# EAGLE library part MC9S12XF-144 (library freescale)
MC9S12XF512 Source: www.freescale.com .. MC9S12XF512V1RM.pdf
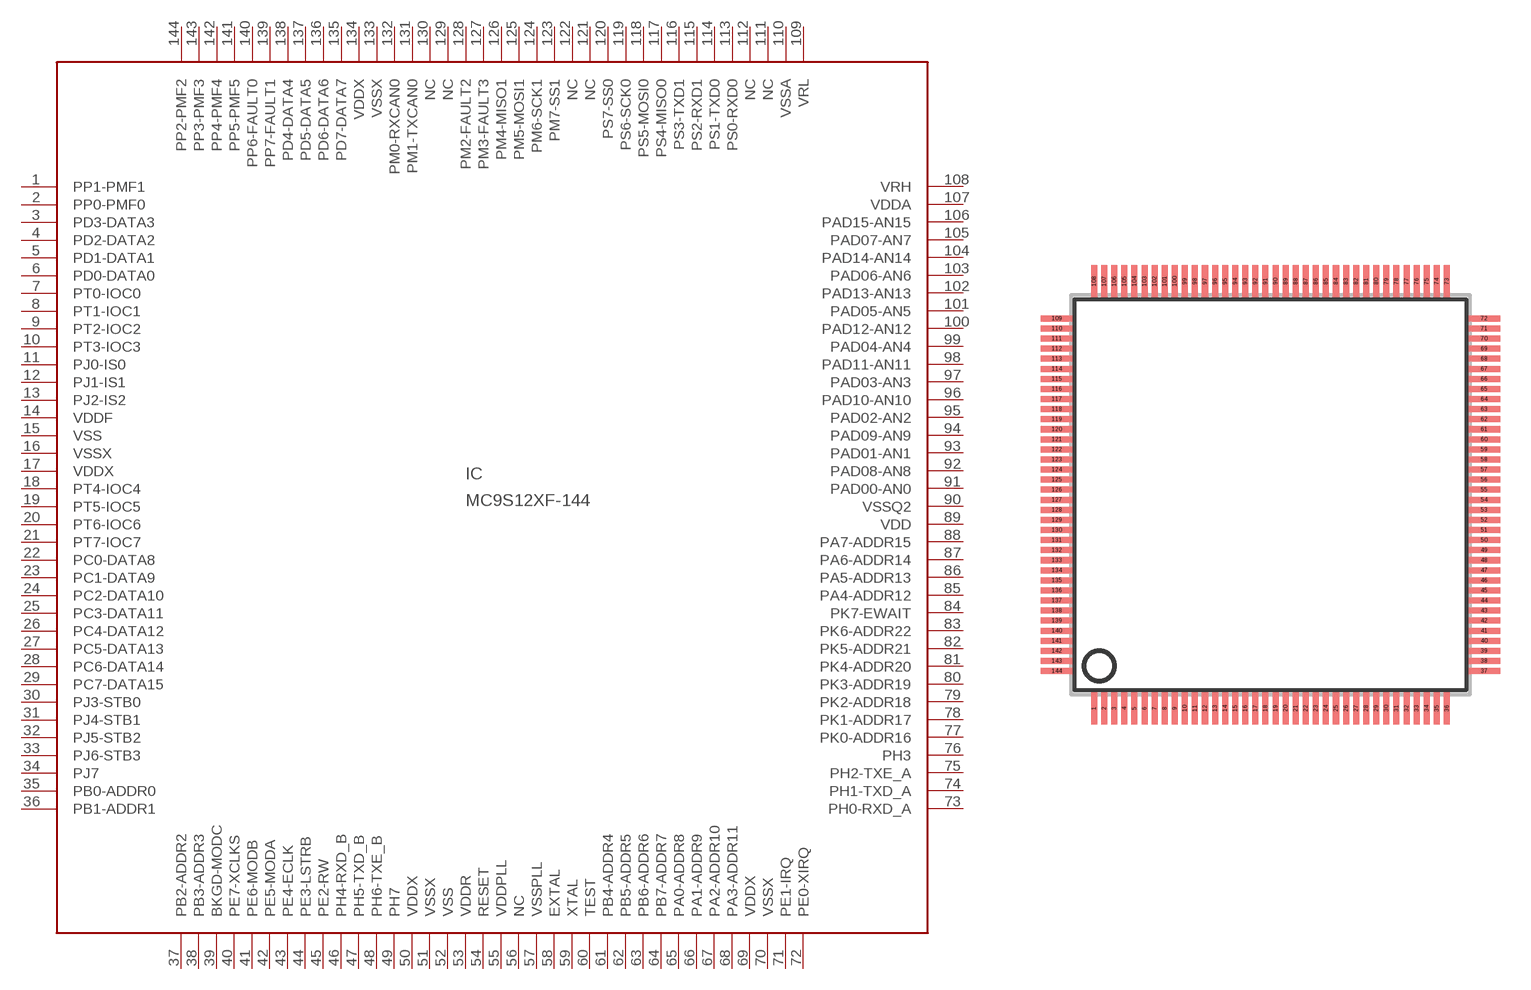
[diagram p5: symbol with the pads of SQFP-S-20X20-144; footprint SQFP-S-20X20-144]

Designator prefix IC

## MC9S12XF-144 (MPN: LFDAS12XFLT; OC_FARNELL: unknown; OC_NEWARK: 14M5920)  [SQFP-S-20X20-144]
1  PP1-PMF1
2  PP0-PMF0
3  PD3-DATA3
4  PD2-DATA2
5  PD1-DATA1
6  PD0-DATA0
7  PT0-IOC0
8  PT1-IOC1
9  PT2-IOC2
10  PT3-IOC3
11  PJ0-IS0
12  PJ1-IS1
13  PJ2-IS2
14  VDDF  pwr
15  VSS  pwr
16  VSSX  pwr
17  VDDX  pwr
18  PT4-IOC4
19  PT5-IOC5
20  PT6-IOC6
21  PT7-IOC7
22  PC0-DATA8
23  PC1-DATA9
24  PC2-DATA10
25  PC3-DATA11
26  PC4-DATA12
27  PC5-DATA13
28  PC6-DATA14
29  PC7-DATA15
30  PJ3-STB0
31  PJ4-STB1
32  PJ5-STB2
33  PJ6-STB3
34  PJ7
35  PB0-ADDR0
36  PB1-ADDR1
37  PB2-ADDR2
38  PB3-ADDR3
39  BKGD-MODC
40  PE7-XCLKS
41  PE6-MODB
42  PE5-MODA
43  PE4-ECLK
44  PE3-LSTRB
45  PE2-RW
46  PH4-RXD_B
47  PH5-TXD_B
48  PH6-TXE_B
49  PH7
50  VDDX  pwr
51  VSSX  pwr
52  VSS  pwr
53  VDDR  pwr
54  RESET
55  VDDPLL  pwr
56  NC  nc
57  VSSPLL  pwr
58  EXTAL  pas
59  XTAL  pas
60  TEST  in
61  PB4-ADDR4
62  PB5-ADDR5
63  PB6-ADDR6
64  PB7-ADDR7
65  PA0-ADDR8
66  PA1-ADDR9
67  PA2-ADDR10
68  PA3-ADDR11
69  VDDX  pwr
70  VSSX  pwr
71  PE1-IRQ  in
72  PE0-XIRQ  in
73  PH0-RXD_A
74  PH1-TXD_A
75  PH2-TXE_A
76  PH3
77  PK0-ADDR16
78  PK1-ADDR17
79  PK2-ADDR18
80  PK3-ADDR19
81  PK4-ADDR20
82  PK5-ADDR21
83  PK6-ADDR22
84  PK7-EWAIT
85  PA4-ADDR12
86  PA5-ADDR13
87  PA6-ADDR14
88  PA7-ADDR15
89  VDD  pwr
90  VSSQ2  pwr
91  PAD00-AN0
92  PAD08-AN8
93  PAD01-AN1
94  PAD09-AN9
95  PAD02-AN2
96  PAD10-AN10
97  PAD03-AN3
98  PAD11-AN11
99  PAD04-AN4
100  PAD12-AN12
101  PAD05-AN5
102  PAD13-AN13
103  PAD06-AN6
104  PAD14-AN14
105  PAD07-AN7
106  PAD15-AN15
107  VDDA  pwr
108  VRH  pwr
109  VRL  pwr
110  VSSA  pwr
111  NC  nc
112  NC  nc
113  PS0-RXD0
114  PS1-TXD0
115  PS2-RXD1
116  PS3-TXD1
117  PS4-MISO0
118  PS5-MOSI0
119  PS6-SCK0
120  PS7-SS0
121  NC  nc
122  NC  nc
123  PM7-SS1
124  PM6-SCK1
125  PM5-MOSI1
126  PM4-MISO1
127  PM3-FAULT3
128  PM2-FAULT2
129  NC  nc
130  NC  nc
131  PM1-TXCAN0
132  PM0-RXCAN0
133  VSSX  pwr
134  VDDX  pwr
135  PD7-DATA7
136  PD6-DATA6
137  PD5-DATA5
138  PD4-DATA4
139  PP7-FAULT1
140  PP6-FAULT0
141  PP5-PMF5
142  PP4-PMF4
143  PP3-PMF3
144  PP2-PMF2

## Footprint SQFP-S-20X20-144 (pad centres in mm)
QFP144 shrink quad flat pack, square
smd 0.3 x 1.6: 1 -8.75,-10.6; 2 -8.25,-10.6; 3 -7.75,-10.6; 4 -7.25,-10.6; 5 -6.75,-10.6; 6 -6.25,-10.6; 7 -5.75,-10.6; 8 -5.25,-10.6; 9 -4.75,-10.6; 10 -4.25,-10.6; 11 -3.75,-10.6; 12 -3.25,-10.6; 13 -2.75,-10.6; 14 -2.25,-10.6; 15 -1.75,-10.6; 16 -1.25,-10.6; 17 -0.75,-10.6; 18 -0.25,-10.6; 19 0.25,-10.6; 20 0.75,-10.6; 21 1.25,-10.6; 22 1.75,-10.6; 23 2.25,-10.6; 24 2.75,-10.6; 25 3.25,-10.6; 26 3.75,-10.6; 27 4.25,-10.6; 28 4.75,-10.6; 29 5.25,-10.6; 30 5.75,-10.6; 31 6.25,-10.6; 32 6.75,-10.6; 33 7.25,-10.6; 34 7.75,-10.6; 35 8.25,-10.6; 36 8.75,-10.6; 73 8.75,10.6; 74 8.25,10.6; 75 7.75,10.6; 76 7.25,10.6; 77 6.75,10.6; 78 6.25,10.6; 79 5.75,10.6; 80 5.25,10.6; 81 4.75,10.6; 82 4.25,10.6; 83 3.75,10.6; 84 3.25,10.6; 85 2.75,10.6; 86 2.25,10.6; 87 1.75,10.6; 88 1.25,10.6; 89 0.75,10.6; 90 0.25,10.6; 91 -0.25,10.6; 92 -0.75,10.6; 93 -1.25,10.6; 94 -1.75,10.6; 95 -2.25,10.6; 96 -2.75,10.6; 97 -3.25,10.6; 98 -3.75,10.6; 99 -4.25,10.6; 100 -4.75,10.6; 101 -5.25,10.6; 102 -5.75,10.6; 103 -6.25,10.6; 104 -6.75,10.6; 105 -7.25,10.6; 106 -7.75,10.6; 107 -8.25,10.6; 108 -8.75,10.6
smd 1.6 x 0.3: 37 10.6,-8.75; 38 10.6,-8.25; 39 10.6,-7.75; 40 10.6,-7.25; 41 10.6,-6.75; 42 10.6,-6.25; 43 10.6,-5.75; 44 10.6,-5.25; 45 10.6,-4.75; 46 10.6,-4.25; 47 10.6,-3.75; 48 10.6,-3.25; 49 10.6,-2.75; 50 10.6,-2.25; 51 10.6,-1.75; 52 10.6,-1.25; 53 10.6,-0.75; 54 10.6,-0.25; 55 10.6,0.25; 56 10.6,0.75; 57 10.6,1.25; 58 10.6,1.75; 59 10.6,2.25; 60 10.6,2.75; 61 10.6,3.25; 62 10.6,3.75; 63 10.6,4.25; 64 10.6,4.75; 65 10.6,5.25; 66 10.6,5.75; 67 10.6,6.25; 68 10.6,6.75; 69 10.6,7.25; 70 10.6,7.75; 71 10.6,8.25; 72 10.6,8.75; 109 -10.6,8.75; 110 -10.6,8.25; 111 -10.6,7.75; 112 -10.6,7.25; 113 -10.6,6.75; 114 -10.6,6.25; 115 -10.6,5.75; 116 -10.6,5.25; 117 -10.6,4.75; 118 -10.6,4.25; 119 -10.6,3.75; 120 -10.6,3.25; 121 -10.6,2.75; 122 -10.6,2.25; 123 -10.6,1.75; 124 -10.6,1.25; 125 -10.6,0.75; 126 -10.6,0.25; 127 -10.6,-0.25; 128 -10.6,-0.75; 129 -10.6,-1.25; 130 -10.6,-1.75; 131 -10.6,-2.25; 132 -10.6,-2.75; 133 -10.6,-3.25; 134 -10.6,-3.75; 135 -10.6,-4.25; 136 -10.6,-4.75; 137 -10.6,-5.25; 138 -10.6,-5.75; 139 -10.6,-6.25; 140 -10.6,-6.75; 141 -10.6,-7.25; 142 -10.6,-7.75; 143 -10.6,-8.25; 144 -10.6,-8.75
